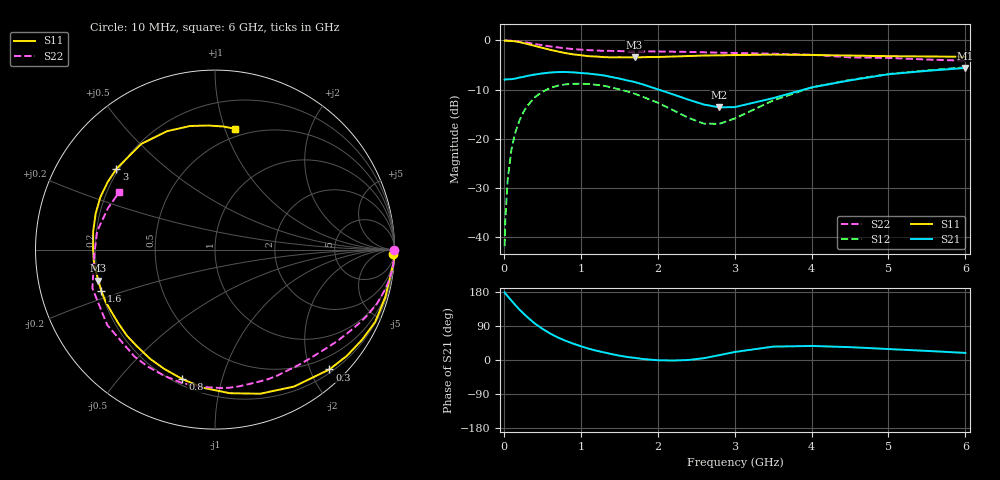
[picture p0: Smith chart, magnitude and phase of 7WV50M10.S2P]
! Infineon Technologies  Discrete & RF Semiconductors
! BFS17W
! Si NPN RF Bipolar Junction Transistor in SOT323
! VCE = 0.5 V  IC = 0.1 mA
! Common Emitter S-Parameters:  August  1999
# GHz  S  MA  R  50
!  f  S11  S21  S12  S22
! GHz  MAG  ANG  MAG  ANG  MAG  ANG  MAG  ANG
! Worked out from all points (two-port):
!   36 points, 10 MHz to 6 GHz, reference 50 ohm
!   highest |S21| = -5.60 dB at 6 GHz (marker M1); lowest = -13.6 dB at 2.8 GHz (marker M2)
!   |S21| within 3 dB of the highest: start of sweep to 1.733 GHz; 4.332 GHz to end of sweep
!   lowest |S11| = -3.4 dB at 1.7 GHz (marker M3), VSWR 5.11, Z = 9.96 - j6.28 ohm
!   |S11| at or under -10 dB: nowhere
!   |S22| runs from -4.1 to 0.0 dB; largest |S21 - S12| = 0.4
!   S11 on the Smith chart (normalised r, x): 10 MHz: 22, -75; 300 MHz: 0.26, -2.31; 800 MHz: 0.23, -0.75; 1.6 GHz: 0.20, -0.17; 3 GHz: 0.19, +0.35; 6 GHz: 0.43, +1.09
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0.01  0.9929 -1.4  0.398 178.5  0.0081 89.7  0.9999 -0.2
0.02  0.9999 -3.4  0.403 175.3  0.0154 85.5  0.9986 -1.3
0.05  0.9889 -7.9  0.403 168.2  0.0386 84.0  0.9977 -3.2
0.1  0.9853 -15.7  0.404 156.5  0.079 79.0  0.9949 -6.5
0.15  0.9793 -24.3  0.41 144.8  0.1165 73.0  0.9851 -9.7
0.2  0.9612 -31.5  0.419 133.7  0.1515 67.8  0.9755 -12.7
0.3  0.9232 -46.3  0.435 114.1  0.2137 57.8  0.9515 -18.4
0.4  0.8811 -60.0  0.45 96.8  0.2635 48.2  0.9227 -23.7
0.5  0.8416 -72.6  0.462 82.5  0.3002 39.8  0.8949 -28.3
0.8  0.7443 -104.1  0.478 50.9  0.3576 20.4  0.8319 -40.8
1.1  0.6924 -128.7  0.461 30.0  0.3609 6.1  0.7977 -52.2
1.6  0.6739 -160.2  0.393 8.0  0.3041 -10.2  0.7751 -71.7
1.7  0.6724 -165.1  0.378 5.7  0.2873 -12.0  0.7727 -75.8
2.2  0.6861 171.6  0.283 -1.4  0.1956 -12.8  0.7691 -95.9
2.6  0.7024 155.4  0.223 4.8  0.1427 5.6  0.7577 -112.0
2.8  0.7064 147.8  0.209 12.7  0.1419 20.7  0.7515 -119.8
3  0.71 140.7  0.21 21.1  0.1607 33.7  0.7462 -126.9
3.5  0.7179 124.9  0.259 35.3  0.2452 45.7  0.7329 -145.0
4  0.7119 112.1  0.333 37.1  0.3329 42.9  0.7161 -162.5
4.5  0.7025 101.3  0.393 33.9  0.397 37.1  0.6731 -177.6
5.5  0.6875 86.0  0.491 24.0  0.4965 25.6  0.6396 158.9
6  0.6818 80.4  0.525 18.7  0.5338 20.3  0.6221 148.8
